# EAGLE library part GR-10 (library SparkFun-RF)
GR-10 GPS Receiver Module Proto layout and schematic for GR-10 GPS receiver. Spark Fun Electronics SKU : GPS-08291
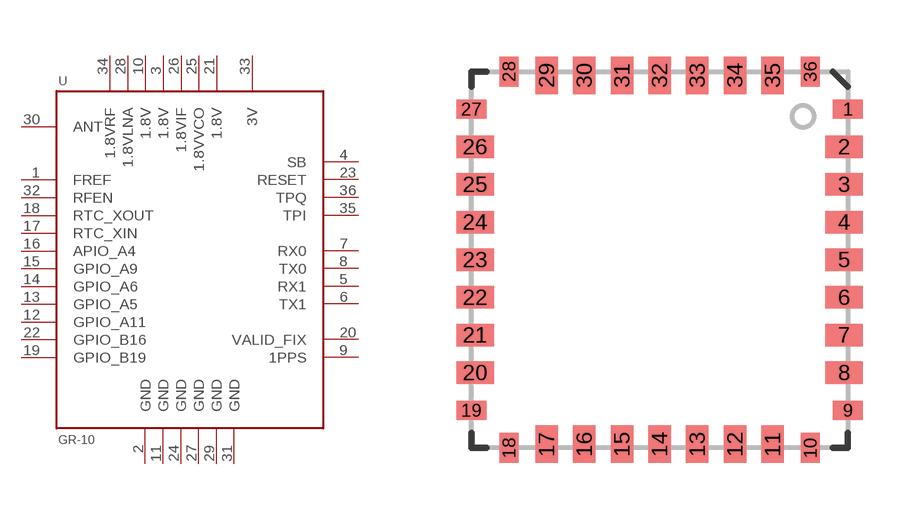
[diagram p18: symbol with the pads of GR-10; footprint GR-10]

Designator prefix -

## GR-10SMD  [GR-10]
1  FREF
2  GND  pwr
3  1.8V  pwr
4  SB  in
5  RX1  in
6  TX1  out
7  RX0  in
8  TX0  out
9  1PPS  out
10  1.8V  pwr
11  GND  pwr
12  GPIO_A11
13  GPIO_A5
14  GPIO_A6
15  GPIO_A9
16  APIO_A4
17  RTC_XIN
18  RTC_XOUT
19  GPIO_B19
20  VALID_FIX  out
21  1.8V  pwr
22  GPIO_B16
23  RESET  in
24  GND  pwr
25  1.8VVCO  pwr
26  1.8VIF  pwr
27  GND  pwr
28  1.8VLNA  pwr
29  GND  pwr
30  ANT  in
31  GND  pwr
32  RFEN  out
33  3V  pwr
34  1.8VRF  pwr
35  TPI  in
36  TPQ  in

## Footprint GR-10 (pad centres in mm)
smd 0.8 x 0.5: 1 5,4; 9 5,-4; 19 -5,-4; 27 -5,4
smd 1 x 0.6: 2 4.9,3; 3 4.9,2; 4 4.9,1; 5 4.9,0; 6 4.9,-1; 7 4.9,-2; 8 4.9,-3; 20 -4.9,-3; 21 -4.9,-2; 22 -4.9,-1; 23 -4.9,0; 24 -4.9,1; 25 -4.9,2; 26 -4.9,3
smd 0.5 x 0.8: 10 4,-5; 18 -4,-5; 28 -4,5; 36 4,5
smd 0.6 x 1: 11 3,-4.9; 12 2,-4.9; 13 1,-4.9; 14 0,-4.9; 15 -1,-4.9; 16 -2,-4.9; 17 -3,-4.9; 29 -3,4.9; 30 -2,4.9; 31 -1,4.9; 32 0,4.9; 33 1,4.9; 34 2,4.9; 35 3,4.9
